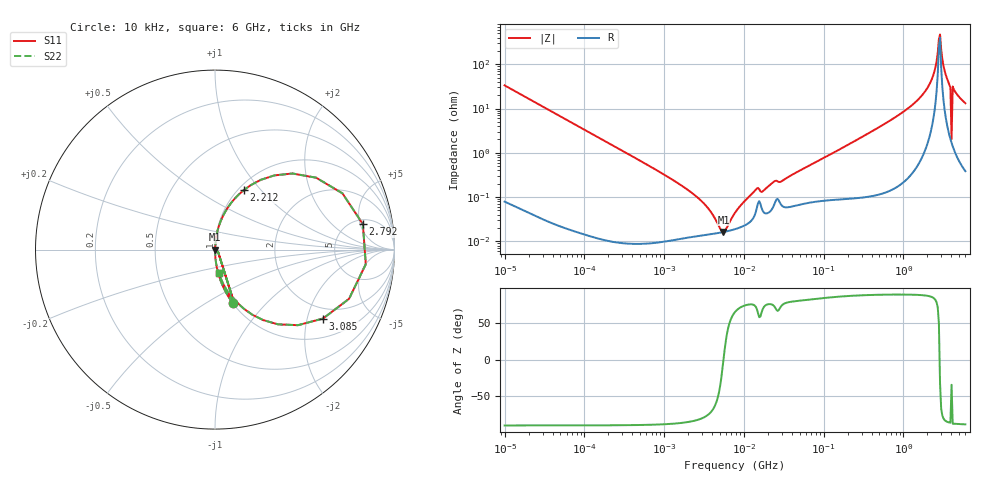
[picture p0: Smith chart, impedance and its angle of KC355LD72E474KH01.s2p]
!Murata Part Number: KC355LD72E474KH01
!These Parameters are Measured in Series Mode Connection
!Data Generated on Jun 19, 2026
!  o--ll--o
!Port1  Port2
!  o------o
!Operation Temp=25[degC], DC Bias Voltage=0[V]
!Freq. Start=10[kHz] Stop=6[GHz] 401[Steps]
# Hz S RI R 50
!Freq.(Hz) S11(Real) S11(Imag) S21(Real) S21(Imag) S12(Real) S12(Imag) S22(Real) S22(Imag)
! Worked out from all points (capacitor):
!   401 points, 10 kHz to 6 GHz, reference 50 ohm
!   read as one part in series: C = 478 nF near 10.69 kHz
!   lowest |Z| = 16.2 mohm at 5.554 MHz (marker M1)
!   series resonance near 5.557 MHz, so ESL is about 1.7 nH
!   S11 on the Smith chart (normalised r, x): 10 kHz: 1.00, -0.67; 2.212 GHz: 1.06, +0.81; 2.792 GHz: 5.88, +5.55; 3.085 GHz: 1.60, -2.51; 6 GHz: 1.01, -0.26
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10000  0.1004 -0.2994  0.8996 0.2994  0.8996 0.2994  0.1004 -0.2994
92862  0.00144 -0.0359  0.9986 0.0359  0.9986 0.0359  0.00144 -0.0359
862344  0.000109 -0.00376  0.9999 0.00376  0.9999 0.00376  0.000109 -0.00376
2855711  0.000135 -0.000844  0.9999 0.000844  0.9999 0.000844  0.000135 -0.000844
5554204  0.000162 -6e-07  0.9998 6e-07  0.9998 6e-07  0.000162 -6e-07
7745967  0.000188 0.000399  0.9998 -0.000399  0.9998 -0.000399  0.000188 0.000399
1.409589e7  0.000455 0.00139  0.9995 -0.00139  0.9995 -0.00139  0.000455 0.00139
1.720936e7  0.000493 0.00125  0.9995 -0.00125  0.9995 -0.00125  0.000493 0.00125
2.40004e7  0.000673 0.00214  0.9993 -0.00214  0.9993 -0.00214  0.000673 0.00214
7.193098e7  0.000793 0.0055  0.9992 -0.0055  0.9992 -0.0055  0.000793 0.0055
6.67969e8  0.00408 0.052  0.9959 -0.052  0.9959 -0.052  0.00408 0.052
1.435489e9  0.0239 0.138  0.9761 -0.138  0.9761 -0.138  0.0239 0.138
2.212024e9  0.1606 0.3316  0.8394 -0.3316  0.8394 -0.3316  0.1606 0.3316
2.526803e9  0.4323 0.424  0.5677 -0.424  0.5677 -0.424  0.4323 0.424
2.791949e9  0.8238 0.1421  0.1762 -0.1421  0.1762 -0.1421  0.8238 0.1421
3.084918e9  0.6018 -0.3841  0.3982 0.3841  0.3982 0.3841  0.6018 -0.3841
3.297118e9  0.3514 -0.4163  0.6486 0.4163  0.6486 0.4163  0.3514 -0.4163
3.643096e9  0.1627 -0.3312  0.8373 0.3312  0.8373 0.3312  0.1627 -0.3312
3.766309e9  0.1276 -0.2994  0.8724 0.2994  0.8724 0.2994  0.1276 -0.2994
4.302268e9  0.0762 -0.2441  0.9238 0.2441  0.9238 0.2441  0.0762 -0.2441
4.447775e9  0.0633 -0.2232  0.9367 0.2232  0.9367 0.2232  0.0633 -0.2232
6e9  0.0206 -0.1283  0.9794 0.1283  0.9794 0.1283  0.0206 -0.1283
